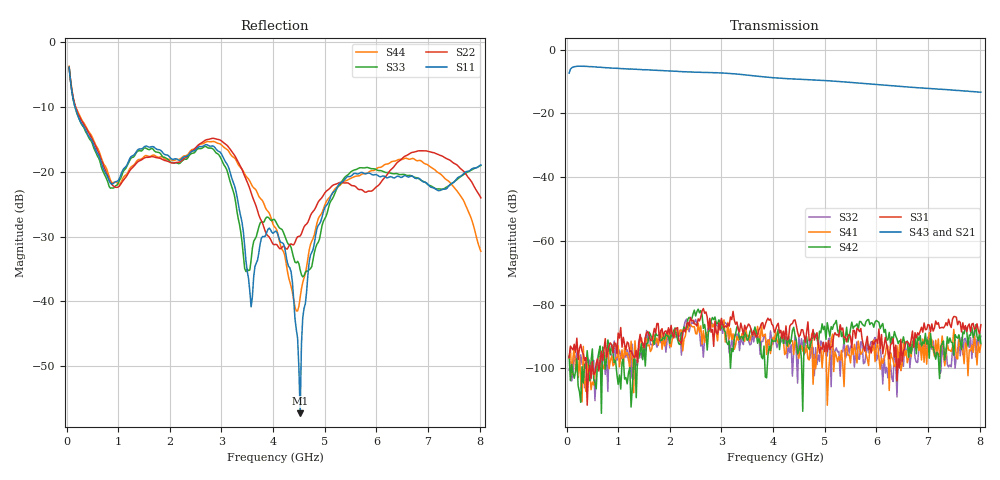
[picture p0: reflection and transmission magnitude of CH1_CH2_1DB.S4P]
!Agilent Technologies,E5071C,MY46316741,A.11.02
!Date: Thu May 28 14:25:44 2026
!Data & Calibration Information:
!1:CH1 INPUT 2:CH1 OUTPUT 3:CH2 INPUT 4:CH2 OUTPUT
!Freq	S11:SOLT4(ON)	S12:SOLT4(ON)	S13:SOLT4(ON)	S14:SOLT4(ON)
!	S21:SOLT4(ON)	S22:SOLT4(ON)	S23:SOLT4(ON)	S24:SOLT4(ON)
!	S31:SOLT4(ON)	S32:SOLT4(ON)	S33:SOLT4(ON)	S34:SOLT4(ON)
!	S41:SOLT4(ON)	S42:SOLT4(ON)	S43:SOLT4(ON)	S44:SOLT4(ON)
!PortZ  Port1:50+j0  Port2:50+j0  Port3:50+j0  Port4:50+j0
!Above PortZ is port z conversion or system Z0 setting when saving the data.
!When reading, reference impedance value at option line is always used.
# Hz S dB R 50
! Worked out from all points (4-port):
!   320 points, 50 MHz to 8.025 GHz, reference 50 ohm
!   strongest paths, dB at 50 MHz, 2.05 GHz, 4.05 GHz, 6.05 GHz, 8.025 GHz:
!     S43: -7.3, -6.7, -8.8, -11.0, -13.3
!     S21: -7.4, -6.8, -8.9, -11.0, -13.4
!     S31: -96.7, -89.5, -87.9, -87.7, -86.3
!     S42: -96.1, -90.2, -91.5, -85.5, -92.3
!     S41: -96.8, -90.7, -88.5, -96.6, -92.7
!     S32: -100.5, -88.8, -91.2, -93.9, -89.9
!   lowest |S11| = -57.3 dB at 4.525 GHz (marker M1), VSWR 1.00, Z = 50 + j0.133 ohm
!   |S11| at or under -10 dB: 165.5 MHz to end of sweep
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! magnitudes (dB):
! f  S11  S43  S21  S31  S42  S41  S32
! 50 MHz  -3.8  -7.3  -7.4  -96.7  -96.1  -96.8  -100.5
! 3 GHz  -17.2  -7.3  -7.4  -84.3  -87.6  -86.2  -86.7
! 3.575 GHz  -40.8  -8.1  -8.2  -87.9  -87.7  -89.7  -92.4
! 4.075 GHz  -29.3  -8.9  -8.9  -86.5  -89.8  -91.1  -93.5
! 4.525 GHz  -57.3  -9.3  -9.4  -89.5  -92.7  -93.6  -95.4
! 5.15 GHz  -23.3  -9.8  -9.9  -93.1  -87.8  -89.3  -90.5
! 8.025 GHz  -18.9  -13.3  -13.4  -86.3  -92.3  -92.7  -89.9
